PROGRAM MAIN
VAR
	//input
	move_up AT%I* : BOOL;                     //上行按钮
    move_down AT%I* : BOOL;                   //下行按钮
	limit_switch_up AT%I*:BOOL;               //上限位
	limit_switch_down AT%I*:BOOL;             //下限位
	//output
	solenoid_valve_up AT%Q*:BOOL;             //上行电磁阀
	solenoid_valve_down AT%Q*:BOOL;           //下行电磁阀
END_VAR

IF move_down THEN  
   solenoid_valve_down:=TRUE;                 //控制下行电磁阀吸合，气缸下行 
   solenoid_valve_up:=FALSE;                                                                                 
END_IF
IF limit_switch_down=TRUE THEN                //触发下限位，下行电磁阀松开
   solenoid_valve_down:=FALSE;  
END_IF


IF move_up THEN   
   solenoid_valve_up:=TRUE;                   //控制上行电磁阀吸合，气缸上行  
solenoid_valve_down:=FALSE;                                                                                        
END_IF

IF limit_switch_up=TRUE THEN                  //触发上限位，上行电磁阀松开
   solenoid_valve_up:=FALSE; 
END_IF

END_PROGRAM
